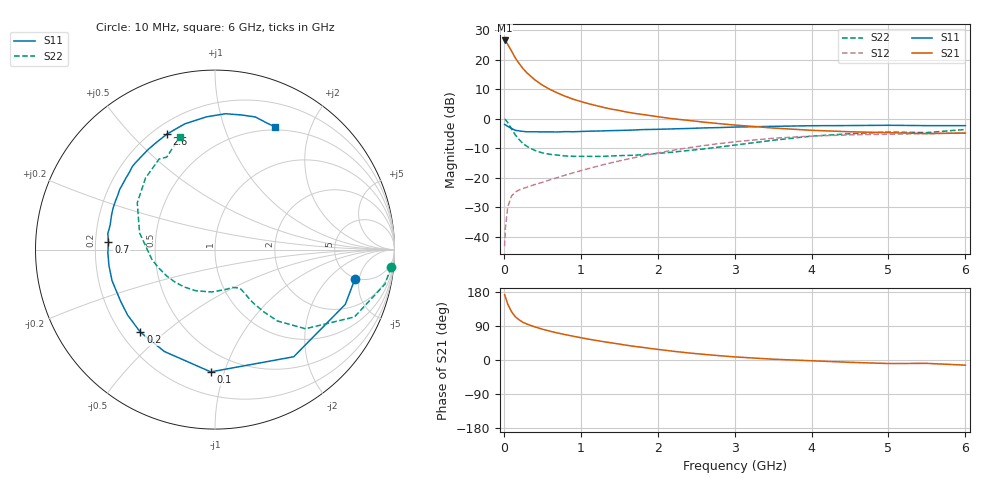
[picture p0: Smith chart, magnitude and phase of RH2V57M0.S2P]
! SIEMENS Small Signal Semiconductors
! BFR106
! Si NPN RF Bipolar Junction Transistor in SOT23
! VCE = 2.5 V  IC = 7 mA
! Common Emitter S-Parameters:  August  1996
# GHz  S  MA  R  50
!  f  S11  S21  S12  S22
! GHz  MAG  ANG  MAG  ANG  MAG  ANG  MAG  ANG
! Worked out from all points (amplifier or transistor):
!   36 points, 10 MHz to 6 GHz, reference 50 ohm
!   highest |S21| = 26.5 dB at 10 MHz (marker M1)
!   |S21| within 3 dB of that: start of sweep to 87.09 MHz
!   unconditionally stable (mu >= 1): 543.7 MHz to 2.179 GHz; 4.674 GHz to end of sweep
!   at 250 MHz: K = 0.60, MSG = 20.3 dB, |S12| = -23.7 dB
!   at 1.4 GHz: K = 1.13, MAG = 6.9 dB, |S12| = -14.9 dB
!   at 6 GHz: K = 1.02, MAG = -0.9 dB, |S12| = -4.7 dB
!   S11 on the Smith chart (normalised r, x): 10 MHz: 4.87, -4.34; 100 MHz: 0.35, -0.90; 200 MHz: 0.28, -0.42; 700 MHz: 0.25, +0.03; 2.6 GHz: 0.25, +0.64; 6 GHz: 0.46, +1.50
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0.01  0.7967 -11.8  21.17 172.2  0.0069 85.3  0.9861 -5.7
0.02  0.7875 -22.8  20.66 166.2  0.0138 80.3  0.9661 -11.5
0.05  0.7408 -53.7  18.22 147.8  0.0318 64.4  0.8626 -25.8
0.1  0.6817 -92.0  14 127.4  0.0489 50.6  0.6694 -41.2
0.15  0.6339 -116.4  10.66 113.9  0.0571 43.1  0.5285 -48.8
0.2  0.6202 -132.1  8.566 105.8  0.0621 41.0  0.4409 -51.9
0.25  0.6084 -143.2  7.041 99.3  0.0656 40.5  0.3771 -54.0
0.3  0.5995 -151.3  5.971 94.8  0.069 41.3  0.3397 -55.0
0.4  0.5992 -163.3  4.585 87.6  0.0763 43.6  0.2904 -55.9
0.5  0.5975 -171.5  3.709 81.4  0.0833 46.3  0.2631 -56.9
0.6  0.5972 -178.4  3.132 76.0  0.0919 49.2  0.249 -59.1
0.7  0.5949 176.0  2.718 71.2  0.1008 51.6  0.2408 -61.8
0.9  0.5999 166.8  2.145 62.8  0.1207 54.9  0.2304 -67.4
1.1  0.6129 158.1  1.796 55.1  0.1424 57.0  0.2297 -76.0
1.3  0.621 150.7  1.547 48.2  0.1668 57.9  0.2298 -84.6
1.6  0.6367 141.1  1.292 38.8  0.2056 57.7  0.2382 -99.3
2.2  0.6712 123.5  0.995 23.1  0.2922 52.6  0.271 -130.3
2.6  0.6971 112.5  0.873 14.9  0.3503 46.9  0.307 -151.6
3.5  0.7411 93.7  0.694 2.1  0.4654 31.4  0.4303 167.5
4.5  0.7645 78.8  0.6 -6.1  0.5308 13.8  0.5556 134.2
5.5  0.7622 67.7  0.559 -8.9  0.5554 3.0  0.5812 117.6
6  0.7614 64.1  0.57 -13.6  0.5816 -4.6  0.6561 107.4
